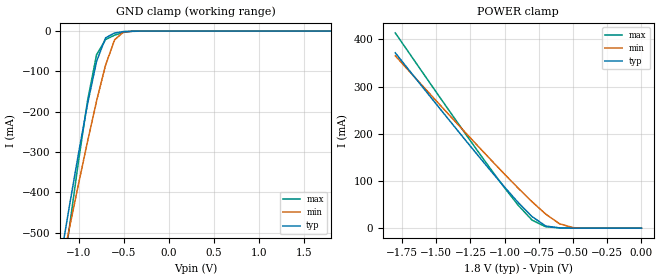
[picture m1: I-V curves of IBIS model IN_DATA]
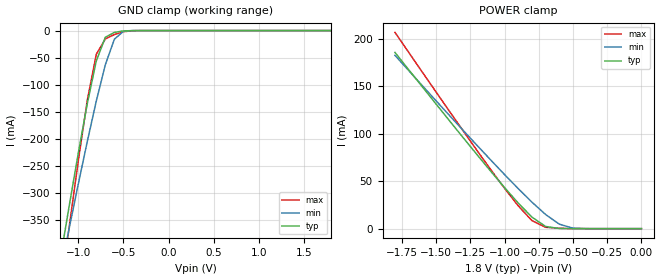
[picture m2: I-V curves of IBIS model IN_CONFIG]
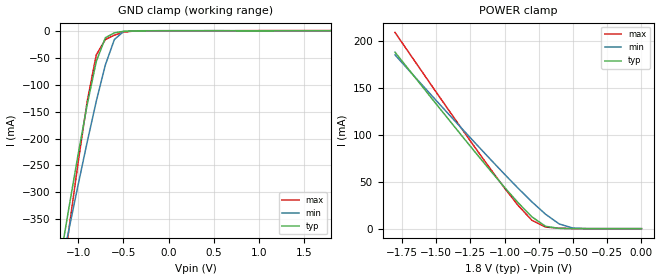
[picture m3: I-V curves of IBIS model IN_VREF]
| IBIS file 4pw864cy_2n.ibs created by s2ibis2 version 1.2
| North Carolina State University Electronics Research Laboratory  1995
[IBIS ver]   2.1
[File name]   4pw864cy_2n.ibs
[File Rev]   1.0
[Date]   Wednesday, October 20, 2004
[Source]   IDT
[Notes]   1. Temp typ=25C, min=0C, max=110C
   2. IDT C11.5 1.8V 1P 2-6M process
   3. Ramp rates based on 500 ohm load
   *** Important Notes ***
[Disclaimer]
READ THESE TERMS AND CONDITIONS CAREFULLY BEFORE USING THIS IBIS MODEL.  BY
USING THIS IBIS MODEL, YOU ARE ACCEPTING AND AGREEING TO THESE TERMS AND
CONDITIONS OF USE.
Integrated Device Technology, Inc. ("IDT") hereby grants the user of this
IBIS model ("User") a non-exclusive, nontransferable license to use this
IBIS model under the following terms: The User is granted this license only
to use the IBIS model for demonstration purposes only and is not granted
rights to sell, copy (except as needed to run the IBIS model), rent, lease
or sub-license (except for demonstration) the IBIS model in whole or in
part, or in modified form to anyone. The User may modify the IBIS model to
suit its specific applications, but  rights to derivative works and such
modifications shall belong to IDT.
THIS IBIS MODEL IS PROVIDED ON AN AS IS" BASIS AND IDT  MAKES ABSOLUTELY NO
WARRANTY WITH RESPECT TO THE INFORMATION CONTAINED HEREIN.  IDT DISCLAIMS
AND USER WAIVES ALL WARRANTIES, EXPRESS AND IMPLIED, INCLUDING WARRANTIES OF
MERCHANTABILITY AND FITNESS FOR A PARTICULAR PURPOSE.  THE ENTIRE RISK AS TO
QUALITY AND PERFORMANCE IS WITH THE USER  ACCORDINGLY, IN NO EVENT SHALL IDT
BE LIABLE FOR ANY DIRECT OR INDIRECT DAMAGES, WHETHER IN CONTRACT OR TORT,
INCLUDING ANY LOST PROFITS OR OTHER INCIDENTAL, CONSEQUENTIAL, EXEMPLARY, OR
PUNITIVE DAMAGES ARISING OUT OF THE USE OR APPLICATION OF THE  IBIS MODEL,
WHETHER OR NOT IDT HAD NOTICE OF SUCH DAMAGES.
IDT reserves the right to make changes without notice to any product herein
to improve reliability, function, or design. IDT does not convey any license
under patent rights or any other intellectual property rights, including
those of third parties. IDT is not obligated to provide  maintenance or
support for the licensed IBIS model.
This model is IDT74SSTU32864C 1:2 Registered Buffer with 1.8 SSTL I/O
[Copyright]
Copyright 2002, Integrated Device Technology, Inc. All rights
reserved.
|   Component IDT4PW864CY
[Component]   IDT4PW864CY
[Manufacturer]   Integrated Device Technology, Inc.
[Package]
|Following package parameters are for 96-pin LFBGA package
| variable   typ   min   max
R_pkg   0.01480   0.01480   0.01480
L_pkg   1.05000nH   1.05000nH   1.05000nH
C_pkg   0.29100pF   0.29100pF   0.29100pF
[Pin]  signal_name   model_name   R_pin   L_pin   C_pin
A1   DCKE/D1   IN_DATA
A2   NC   NC
A3   VREF   IN_VREF
A4   VDD   POWER
A5   QCKEA/Q1A   OUTBUF
A6   QCKEB/Q1B   OUTBUF
B1   D2   IN_DATA
B2   NC   NC
B3   GND   GND
B4   GND   GND
B5   Q2A   OUTBUF
B6   Q2B   OUTBUF
C1   D3   IN_DATA
C2   NC   NC
C3   VDD   POWER
C4   VDD   POWER
C5   Q3A   OUTBUF
C6   Q3B   OUTBUF
D1   DODT/D4   IN_DATA
D2   NC   NC
D3   GND   GND
D4   GND   GND
D5   QODTA/Q4A   OUTBUF
D6   QODTB/Q4B   OUTBUF
E1   D5   IN_DATA
E2   NC   NC
E3   VDD   POWER
E4   VDD   POWER
E5   Q5A   OUTBUF
E6   Q5B   OUTBUF
F1   D6   IN_DATA
F2   NC   NC
F3   GND   GND
F4   GND   GND
F5   Q6A   OUTBUF
F6   Q6B   OUTBUF
G1   NC   NC
G2   _RESET_   IN_RESET
G3   VDD   POWER
G4   VDD   POWER
G5   C1   IN_CONFIG
G6   C0   IN_CONFIG
H1   CLK   IN_CLK
H2   _DCS_   IN_CSGATEN
H3   GND   GND
H4   GND   GND
H5   _QCSA_   OUTBUF
H6   _QCSB_   OUTBUF
J1   _CLK_   IN_CLK
J2   _CSR_   IN_CSGATEN
J3   VDD   POWER
J4   VDD   POWER
J5   NC   NC
J6   NC   NC
K1   D8   IN_DATA
K2   NC   NC
K3   GND   GND
K4   GND   GND
K5   Q8A   OUTBUF
K6   Q8B   OUTBUF
L1   D9   IN_DATA
L2   NC   NC
L3   VDD   POWER
L4   VDD   POWER
L5   Q9A   OUTBUF
L6   Q9B   OUTBUF
M1   D10   IN_DATA
M2   NC   NC
M3   GND   GND
M4   GND   GND
M5   Q10A   OUTBUF
M6   Q10B   OUTBUF
N1   D11/DODT   IN_DATA
N2   NC   NC
N3   VDD   POWER
N4   VDD   POWER
N5   Q11A/QODTA   OUTBUF
N6   Q11B/QODTB   OUTBUF
P1   D12   IN_DATA
P2   NC   NC
P3   GND   GND
P4   GND   GND
P5   Q12A   OUTBUF
P6   Q12B   OUTBUF
R1   D13   IN_DATA
R2   NC   NC
R3   VDD   POWER
R4   VDD   POWER
R5   Q13A   OUTBUF
R6   Q13B   OUTBUF
T1   D14/DCKE   IN_DATA
T2   NC   NC
T3   VREF   IN_VREF
T4   VDD   POWER
T5   Q14A/QCKEA   OUTBUF
T6   Q14B/QCKEB   OUTBUF
| d   d   dummy_model
| din  din   dummy_model
[Diff Pin]  inv_pin   vdiff   tdelay_typ  tdelay_min  tdelay_max
H1   J1   0.60000V  NA   |CLK<P:N> Input  Pair
| Models and submodels in the file (7): IN_DATA (Input), IN_CONFIG (Input), IN_VREF (Input), IN_CLK (Input), IN_CSGATEN (Input), IN_RESET (Input), OUTBUF (Output)
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|   Model IN_DATA
[Model]   IN_DATA
Model_type   Input
Vinl =  0.65000V
Vinh =  1.15000V
C_comp   2.50000pF   2.50000pF   2.50000pF
[Temperature Range]   25.00000   0.11000k   0.000
[Voltage Range]   1.80000V   1.70000V   1.90000V
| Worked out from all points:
|   GND clamp passes 1 mA (typ) near -0.49 V on its own axis
|   POWER clamp passes 1 mA (typ) near -0.61 V on its own axis
[GND_clamp]
| voltage   I(typ)   I(min)   I(max)
-1.8V     -1.39A     -1.277A    -1.696A
-1.2V     -565.7mA   -597.8mA   -652.4mA
-1.1V     -432.9mA   -487.6mA   -484.9mA
-1V       -303.6mA   -379.3mA   -322.8mA
-900mV    -181mA     -273.9mA   -172.7mA
-800mV    -75.14mA   -173.7mA   -58.62mA
-700mV    -16.73mA   -84.3mA    -20.99mA
-600mV    -4.676mA   -21.46mA   -10.1mA
-500mV    -1.061mA   -2.105mA   -3.219mA
-300mV    -27.07uA   -36.06uA   -179.2uA
1.8V      22.11nA    16.44nA    848.8pA
[POWER_clamp]
| voltage   I(typ)   I(min)   I(max)
-1.8V     371.6mA    365.3mA    413.8mA
-1.4V     226.9mA    238.1mA    246.6mA
-1.1V     120.8mA    144.6mA    124.3mA
-900mV    53.98mA    84.46mA    48.22mA
-800mV    24.48mA    55.97mA    17.07mA
-700mV    4.618mA    29.87mA    2.867mA
-600mV    374.6uA    9.474mA    728uA
-500mV    44.79uA    1.038mA    142.2uA
0V        1.16nA     1.231nA    138.3nA
|   Model IN_CONFIG
[Model]   IN_CONFIG
Model_type   Input
Vinl =  0.000V
Vinh =  1.80000V
C_comp   1.750000pF   1.75000pF   1.75000pF
[Temperature Range]   25.00000   0.11000k   0.000
[Voltage Range]   1.80000V   1.70000V   1.90000V
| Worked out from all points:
|   GND clamp passes 1 mA (typ) near -0.51 V on its own axis
|   POWER clamp passes 1 mA (typ) near -0.64 V on its own axis
[GND_clamp]
| voltage   I(typ)   I(min)   I(max)
-1.8V     -1.043A    -959.4mA   -1.273A
-1.2V     -424.5mA   -449mA     -489.5mA
-1.1V     -324.8mA   -366.2mA   -363.7mA
-1V       -227.7mA   -284.8mA   -242.1mA
-900mV    -135.7mA   -205.7mA   -129.5mA
-800mV    -56.25mA   -130.4mA   -43.87mA
-700mV    -12.4mA    -63.21mA   -15.59mA
-600mV    -3.339mA   -15.99mA   -7.372mA
-500mV    -641.5uA   -1.45mA    -2.182mA
-300mV    -2.084uA   -3.939uA   -10.01uA
1.8V      25.37pA    8.201nA    -20.58pA
[POWER_clamp]
| voltage   I(typ)   I(min)   I(max)
-1.8V     185.8mA    182.7mA    206.9mA
-1.4V     113.4mA    119mA      123.3mA
-1.1V     60.42mA    72.28mA    62.15mA
-900mV    26.99mA    42.23mA    24.11mA
-800mV    12.24mA    27.99mA    8.537mA
-700mV    2.309mA    14.93mA    1.433mA
-600mV    187.3uA    4.737mA    363.9uA
-500mV    22.39uA    519.1uA    71.04uA
0V        25.37pA    590pA      7.891pA
|   Model IN_VREF
[Model]   IN_VREF
Model_type   Input
Vinl =  0.83300V
Vinh =  0.96900V
C_comp   1.750000pF   1.75000pF   1.75000pF
[Temperature Range]   25.00000   0.11000k   0.000
[Voltage Range]   1.80000V   1.70000V   1.90000V
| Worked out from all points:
|   GND clamp passes 1 mA (typ) near -0.48 V on its own axis
|   POWER clamp passes 1 mA (typ) near -0.63 V on its own axis
[GND_clamp]
| voltage   I(typ)   I(min)   I(max)
-1.8V     -1.044A    -959.5mA   -1.274A
-1.2V     -425.3mA   -449.2mA   -490.5mA
-1.1V     -325.6mA   -366.4mA   -364.7mA
-1V       -228.5mA   -285.1mA   -243.1mA
-900mV    -136.5mA   -205.9mA   -130.4mA
-800mV    -56.98mA   -130.7mA   -44.72mA
-700mV    -13.07mA   -63.55mA   -16.39mA
-600mV    -3.939mA   -16.32mA   -8.116mA
-500mV    -1.14mA    -1.7mA     -2.847mA
-400mV    -392.1uA   -191.6uA   -763.5uA
-200mV    -76.88uA   -1.393uA   -124uA
1.8V      3.742nA    18.4nA     284.3uA
[POWER_clamp]
| voltage   I(typ)   I(min)   I(max)
-1.8V     187.9mA    185mA      208.9mA
-1.4V     114.8mA    120.6mA    124.6mA
-1.1V     61.24mA    73.34mA    62.99mA
-900mV    27.48mA    42.95mA    24.62mA
-800mV    12.57mA    28.54mA    8.907mA
-700mV    2.495mA    15.32mA    1.676mA
-600mV    263.6uA    4.975mA    490.6uA
-500mV    40.7uA     624.8uA    116.1uA
0V        44.61nA    2.953nA    193.8nA
